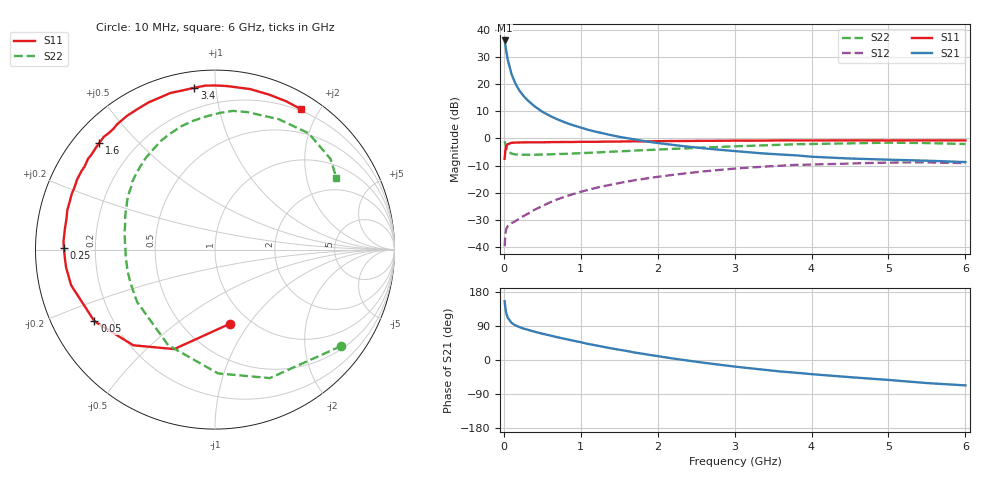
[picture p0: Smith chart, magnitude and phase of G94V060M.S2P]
! SIEMENS Small Signal Semiconductors
! BFG235
! Si NPN RF Bipolar Junction Transistor in SOT223
! VCE = 4 V  IC = 60 mA
! Common Emitter S-Parameters:  July  1994
# GHz  S  MA  R  50
!  f  S11  S21  S12  S22
! GHz  MAG  ANG  MAG  ANG  MAG  ANG  MAG  ANG
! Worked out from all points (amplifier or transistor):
!   40 points, 10 MHz to 6 GHz, reference 50 ohm
!   highest |S21| = 36.0 dB at 10 MHz (marker M1)
!   |S21| within 3 dB of that: start of sweep to 26.52 MHz
!   unconditionally stable (mu >= 1): 479.7 MHz to 1.426 GHz
!   at 200 MHz: K = 0.71, MSG = 23.6 dB, |S12| = -29.6 dB
!   at 1.5 GHz: K = 0.99, MSG = 8.5 dB, |S12| = -16.4 dB
!   at 6 GHz: K = 0.92, MSG = 0.2 dB, |S12| = -9.1 dB
!   S11 on the Smith chart (normalised r, x): 10 MHz: 0.82, -0.82; 50 MHz: 0.13, -0.27; 250 MHz: 0.09, +0.01; 1.6 GHz: 0.08, +0.39; 3.4 GHz: 0.08, +0.88; 6 GHz: 0.18, +1.78
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0.01  0.4208 -78.3  63.01 155.3  0.0104 66.9  0.8847 -37.4
0.02  0.599 -112.3  51.27 137.3  0.0173 51.6  0.7784 -66.9
0.03  0.7012 -130.5  41.41 125.1  0.0213 42.6  0.69 -88.6
0.05  0.7817 -149.3  28.23 111.7  0.0243 33.2  0.5929 -116.1
0.1  0.8259 -166.1  15.13 98.2  0.0275 31.4  0.523 -146.2
0.15  0.8357 -173.3  10.2 91.5  0.03 35.6  0.5058 -159.0
0.2  0.8383 -177.3  7.641 87.1  0.0332 39.4  0.5016 -166.2
0.25  0.8422 179.3  6.16 83.3  0.0368 43.1  0.4987 -171.0
0.3  0.8452 176.9  5.139 80.4  0.0402 46.3  0.4987 -174.9
0.4  0.8443 172.1  3.87 74.6  0.0486 50.3  0.4994 179.7
0.5  0.8451 168.3  3.091 69.4  0.057 52.6  0.5033 175.5
0.6  0.8515 165.1  2.582 64.8  0.0663 53.6  0.5081 171.7
0.7  0.8526 161.4  2.224 59.9  0.0759 54.1  0.5138 168.4
0.9  0.8562 155.9  1.741 51.1  0.0942 52.7  0.5253 162.5
1.1  0.863 149.7  1.426 42.2  0.1133 50.4  0.5415 156.7
1.6  0.8773 137.2  1.008 23.7  0.1599 41.7  0.5832 143.2
2.2  0.8921 123.4  0.756 3.9  0.2131 29.3  0.6401 127.0
3.2  0.9049 101.6  0.552 -21.8  0.2903 5.9  0.7277 99.6
3.4  0.9092 97.3  0.524 -26.1  0.3023 1.0  0.7437 93.7
4.5  0.9156 77.6  0.425 -45.3  0.3438 -24.7  0.8089 63.9
5.5  0.9166 64.4  0.388 -60.9  0.361 -46.8  0.8181 38.1
6  0.9174 58.4  0.366 -67.0  0.3503 -55.1  0.7857 30.7
